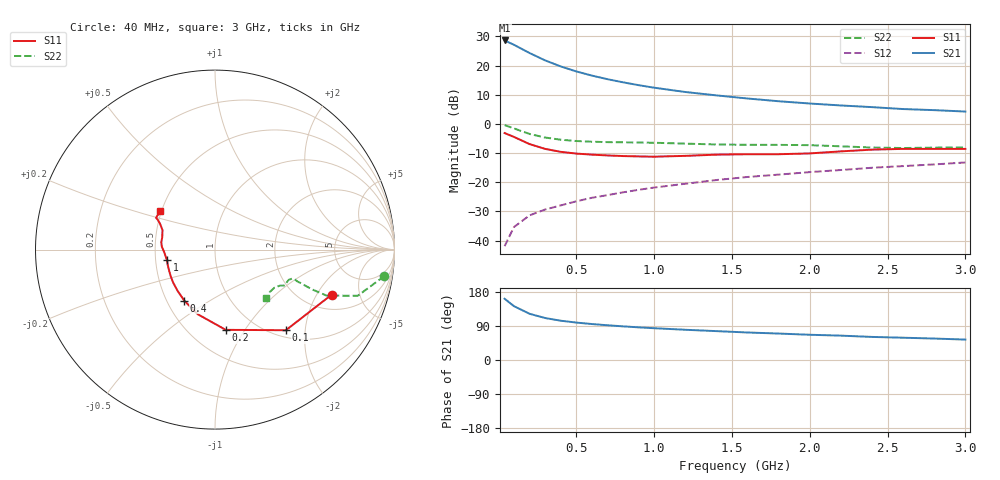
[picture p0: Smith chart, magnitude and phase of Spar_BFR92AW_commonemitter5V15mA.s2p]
! Filename:  BFR92AWD.S2P  Version:  4.0
! NXP part #: BFR92AW  Date: Jun 1994
! Bias condition: Vce=5V, Ic=15mA
#  MHz  S  MA  R  50
! Freq  S11  S21  S12  S22  !GUM [dB]
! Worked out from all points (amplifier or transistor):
!   21 points, 40 MHz to 3 GHz, reference 50 ohm
!   highest |S21| = 28.6 dB at 40 MHz (marker M1)
!   |S21| within 3 dB of that: start of sweep to 153.7 MHz
!   unconditionally stable (mu >= 1): 588.8 MHz to end of sweep
!   at 300 MHz: K = 0.78, MSG = 25.6 dB, |S12| = -29.4 dB
!   at 1 GHz: K = 1.10, MAG = 15.2 dB, |S12| = -21.8 dB
!   at 3 GHz: K = 1.07, MAG = 7.1 dB, |S12| = -13.2 dB
!   lowest NFmin = 2.30 dB at 500 MHz
!   S11 on the Smith chart (normalised r, x): 40 MHz: 2.78, -2.71; 100 MHz: 1.13, -1.58; 200 MHz: 0.73, -0.82; 400 MHz: 0.61, -0.39; 1 GHz: 0.57, -0.07; 3 GHz: 0.49, +0.25
40  0.697 -21.1  26.99 161.6  0.008 80.8  0.955 -8.9
100  0.598 -48.7  22.75 142.1  0.017 69.6  0.836 -17.9
200  0.451 -82.4  16.44 122.0  0.027 63.4  0.673 -22.4
300  0.373 -104.8  12.29 110.8  0.034 62.6  0.584 -22.3
400  0.332 -121.0  9.684 103.7  0.04 64.8  0.536 -21.7
500  0.31 -132.4  7.95 98.8  0.047 66.5  0.509 -21.3
600  0.297 -141.7  6.748 94.9  0.054 68.4  0.495 -21.2
700  0.288 -149.0  5.851 91.7  0.06 69.8  0.487 -21.0
800  0.281 -155.6  5.172 88.8  0.067 70.9  0.484 -20.9
900  0.277 -161.8  4.623 86.2  0.074 71.8  0.48 -20.6
1000  0.274 -167.5  4.18 83.9  0.081 72.7  0.475 -20.5
1200  0.283 -176.9  3.526 79.8  0.094 73.7  0.459 -20.6
1400  0.297 176.7  3.086 76.2  0.109 74.4  0.444 -22.3
1600  0.302 172.2  2.728 72.6  0.123 74.8  0.438 -25.2
1800  0.302 166.7  2.448 69.8  0.135 75.4  0.437 -26.9
2000  0.312 159.7  2.238 66.6  0.149 75.8  0.432 -27.7
2200  0.338 154.8  2.072 64.3  0.162 76.1  0.413 -29.1
2400  0.362 152.3  1.94 60.9  0.177 76.1  0.393 -32.7
2600  0.373 151.7  1.798 58.8  0.189 75.9  0.386 -37.8
2800  0.373 149.3  1.722 56.6  0.202 76.4  0.392 -41.4
3000  0.373 144.9  1.629 53.9  0.218 76.4  0.395 -43.6
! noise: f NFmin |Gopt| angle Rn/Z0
500  2.3  0.222  25.2  0.332
1000  2.8  0.151  66.2  0.37
2000  3.7  0.222  -164.7  0.3
